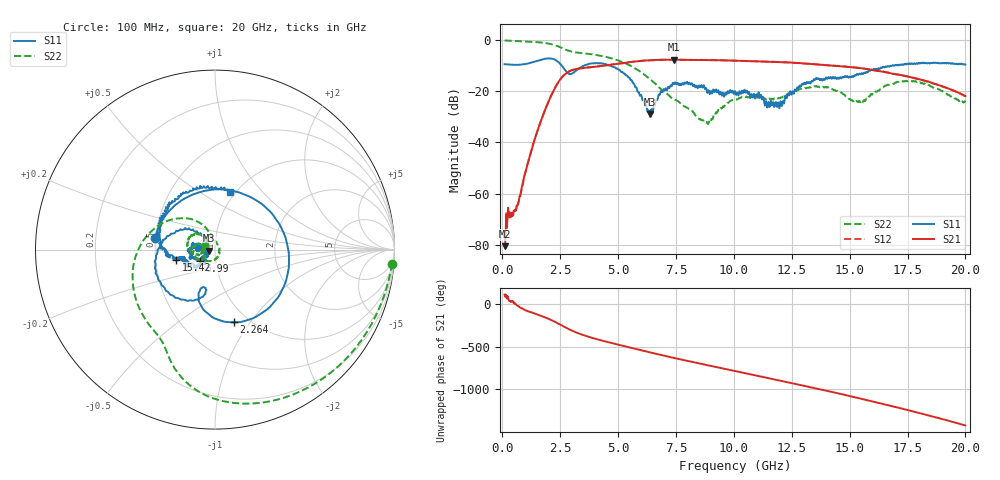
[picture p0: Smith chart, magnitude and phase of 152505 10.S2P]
!  2-Port S-parameters saved by WinCal
! VAR MeasName=S-Parameters (CALIBRATED_DATA) read from VNA (N5230C)
! VAR MeasDate=4/10/2015 9:29:19 AM
! VAR NAME=152505 10
! VAR FILENAME=152505 10.S2P
! VAR DATE=4/10/2015 9:29:19 AM
! VAR PHYS_PORTS=1,2
# Hz S DB R 50
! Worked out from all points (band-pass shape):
!   801 points, 100 MHz to 20 GHz, reference 50 ohm
!   highest |S21| = -7.62 dB at 7.413 GHz (marker M1); lowest = -80.6 dB at 100 MHz (marker M2)
!   |S21| within 3 dB of the highest: 3.736 GHz to 15.14 GHz (11.4 GHz wide, 121 % of centre)
!   lowest |S11| = -28.8 dB at 6.393 GHz (marker M3), VSWR 1.08, Z = 46.6 - j0.63 ohm
!   |S11| at or under -10 dB: 2.571 GHz to 3.52 GHz (949.6 MHz wide, 31.2 % of centre); 4.689 GHz to 16.76 GHz (12.07 GHz wide, 113 % of centre); 16.78154 GHz to 16.82571 GHz (44.18 MHz wide, 0.263 % of centre)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
!   |S22| runs from -32.8 to -0.1 dB; largest |S21 - S12| = 0.0063
!   S11 on the Smith chart (normalised r, x): 100 MHz: 0.50, +0.07; 2.264 GHz: 0.86, -0.84; 6.99 GHz: 0.84, -0.11; 15.42 GHz: 0.64, -0.08; 20 GHz: 0.94, +0.69
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1e8  -9.38 168.8  -80.56 105.8  -74.89 140.1  -0.08 -4.6
2.74125e8  -9.48 149.6  -67.28 43.4  -66.92 46.8  -0.17 -11.5
6.22375e8  -9.61 112.1  -64.84 -17.3  -64.61 -16.8  -0.30 -25.3
1.04525e9  -9.22 66.0  -50.07 -81.7  -50.11 -81.5  -0.47 -42.3
1.716875e9  -7.53 -11.1  -30.32 -146.0  -30.35 -145.8  -0.93 -70.5
2.264125e9  -7.57 -75.4  -18.84 149.3  -18.84 149.5  -1.90 -95.4
2.886e9  -13.23 -107.8  -12.20 61.2  -12.18 61.4  -4.16 -116.4
3.43325e9  -10.36 -111.9  -10.95 -0.4  -10.92 -0.2  -5.03 -129.5
4.82625e9  -10.59 171.8  -9.41 -106.0  -9.37 -106.0  -7.37 -179.7
5.5725e9  -15.60 137.2  -8.49 -155.2  -8.46 -155.4  -10.15 149.2
6.393375e9  -28.81 -169.3  -7.81 151.3  -7.82 151.3  -15.30 119.7
6.741625e9  -21.55 -151.1  -7.69 129.2  -7.67 128.9  -18.15 111.8
6.990375e9  -19.51 -143.5  -7.65 113.4  -7.66 113.4  -20.05 107.5
7.41325e9  -17.20 -160.1  -7.62 87.9  -7.61 87.8  -23.11 104.6
8.880875e9  -20.21 166.6  -7.75 1.8  -7.75 1.8  -32.80 -5.4
1.005e10  -19.91 -177.6  -7.97 -65.3  -7.99 -65.6  -23.23 -110.0
1.1841e10  -25.39 -148.1  -8.47 -167.6  -8.53 -167.8  -22.77 -142.9
1.338325e10  -16.03 -146.6  -9.34 101.7  -9.27 101.9  -18.11 -165.3
1.5423e10  -13.04 -165.5  -10.85 -23.3  -10.85 -24.0  -23.73 -175.1
1.669162e10  -10.28 173.5  -12.74 -105.5  -12.80 -106.8  -17.46 -173.9
1.853238e10  -8.90 124.4  -16.59 128.6  -16.79 128.1  -18.08 136.4
2e10  -9.52 75.3  -21.87 20.9  -21.92 21.3  -24.16 160.2
